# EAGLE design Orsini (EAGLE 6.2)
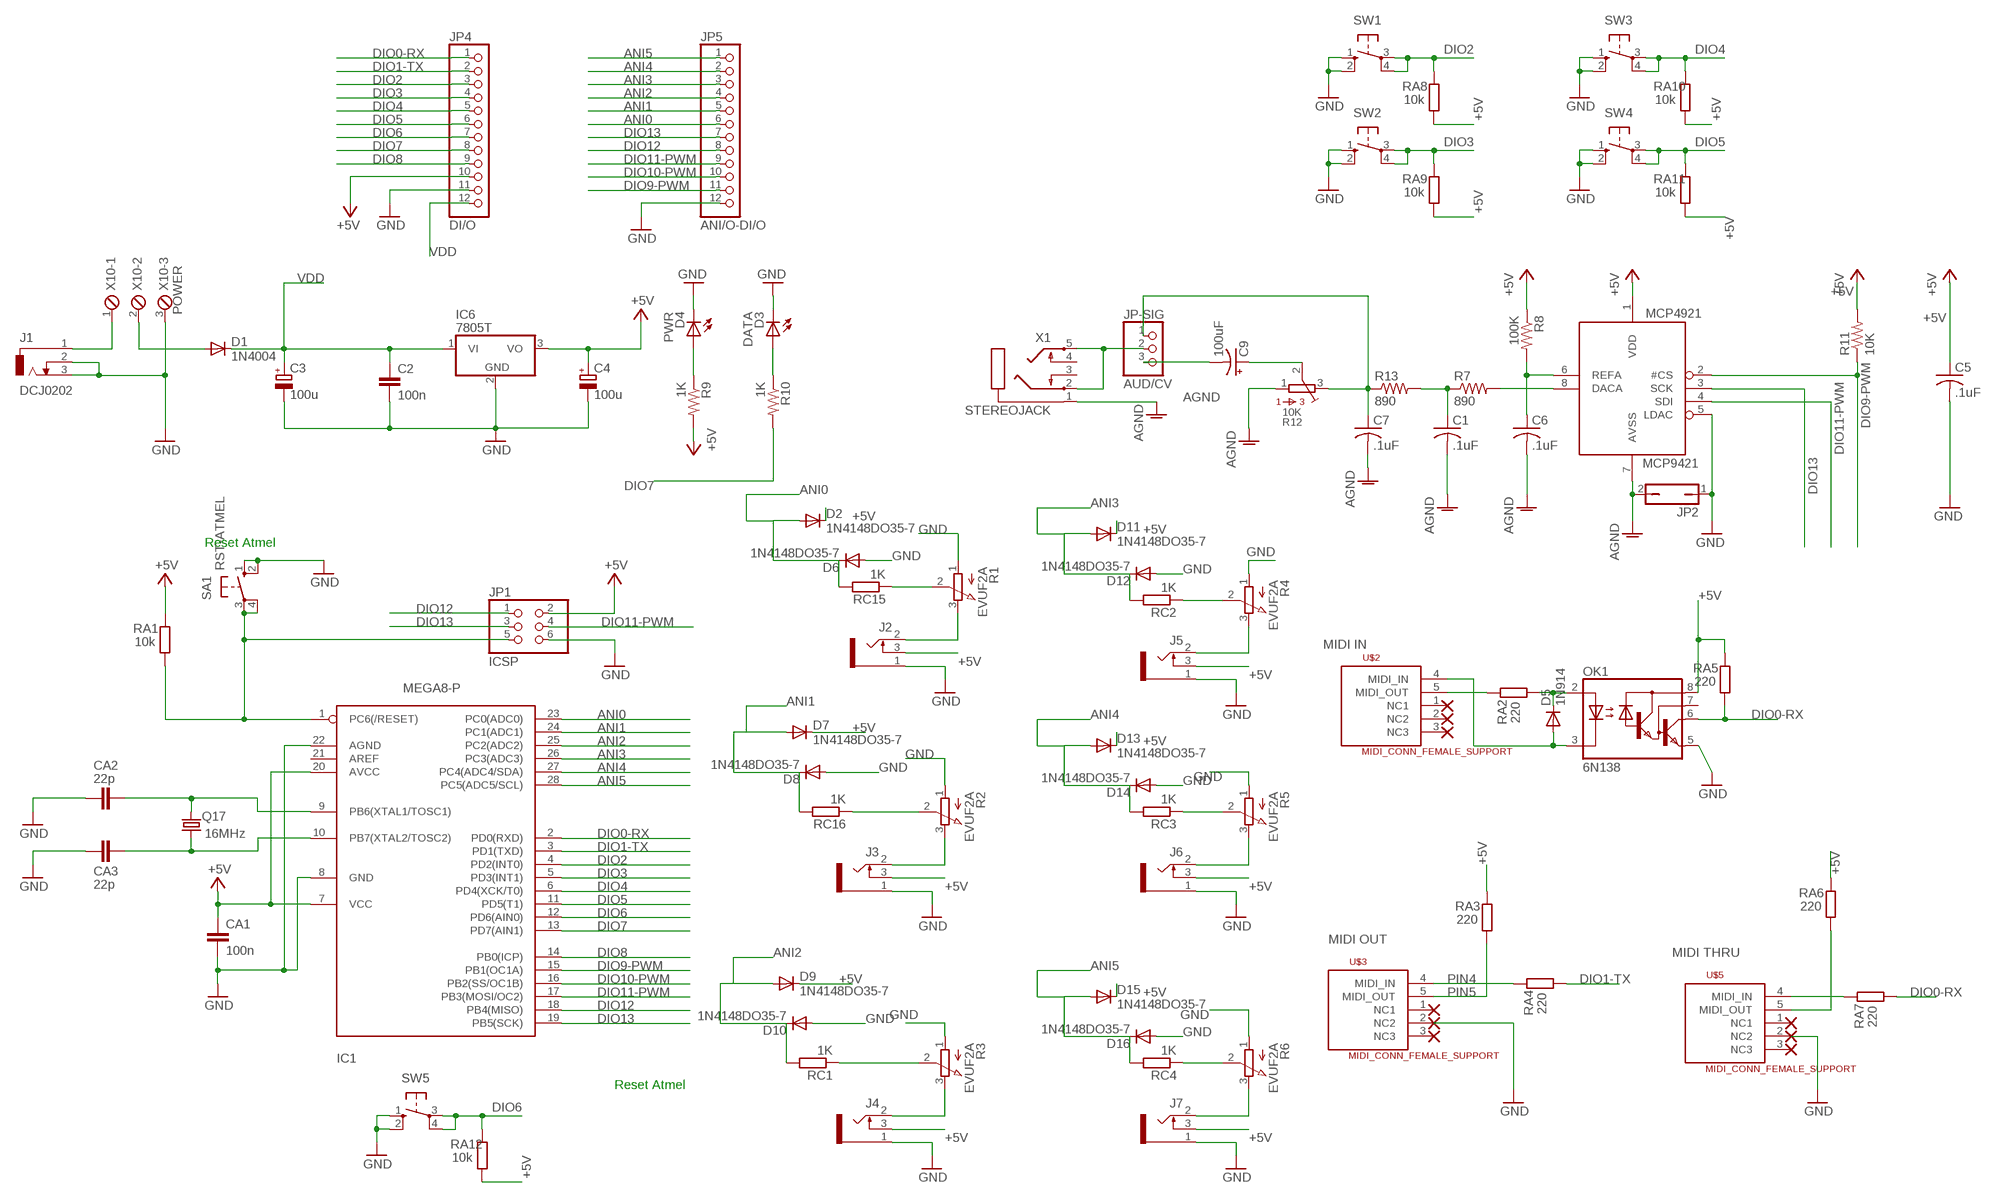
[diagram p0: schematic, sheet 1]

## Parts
C1  .1uF  C-US050-025X075  [C050-025X075]
C2  100n  C-EU050-025X075  [C050-025X075]
C3  100u  CPOL-EUE2.5-7  [E2,5-7]
C4  100u  CPOL-EUE2.5-7  [E2,5-7]
C5  .1uF  C-US025-025X050  [C025-025X050]
C6  .1uF  C-US025-025X050  [C025-025X050]
C7  .1uF  C-US050-025X075  [C050-025X075]
C9  100uF  CPOL-USE2.5-5  [E2,5-5]
CA1  100n  C-EU050-025X075  [C050-025X075]
CA2  22p  C-EU050-025X075  [C050-025X075]
CA3  22p  C-EU050-025X075  [C050-025X075]
D1  1N4004  [DO41-10]
D2  1N4148DO35-7  [DO35-7]
D3  DATA  HLMP-M  [LED4MM]
D4  PWR  HLMP-M  [LED4MM]
D5  1N914  BAS15  [DO34-7]
D6  1N4148DO35-7  [DO35-7]
D7  1N4148DO35-7  [DO35-7]
D8  1N4148DO35-7  [DO35-7]
D9  1N4148DO35-7  [DO35-7]
D10  1N4148DO35-7  [DO35-7]
D11  1N4148DO35-7  [DO35-7]
D12  1N4148DO35-7  [DO35-7]
D13  1N4148DO35-7  [DO35-7]
D14  1N4148DO35-7  [DO35-7]
D15  1N4148DO35-7  [DO35-7]
D16  1N4148DO35-7  [DO35-7]
IC1  MEGA8-P  [DIL28-3]
IC6  7805T  [TO220H]
J1  DCJ0202  [DCJ0202]
J2  1502_03SLOTTED  [1502_03_SLOTTED]
J3  1502_03SLOTTED  [1502_03_SLOTTED]
J4  1502_03SLOTTED  [1502_03_SLOTTED]
J5  1502_03SLOTTED  [1502_03_SLOTTED]
J6  1502_03SLOTTED  [1502_03_SLOTTED]
J7  1502_03SLOTTED  [1502_03_SLOTTED]
JP1  ICSP  PINHD-2X3  [2X03]
JP2  JP1Q  [JP1]
JP4  DI/O  PINHD-1X12  [1X12]
JP5  ANI/O-DI/O  PINHD-1X12  [1X12]
JP-SIG  AUD/CV  PINHD-1X3  [1X03]
MCP4921  MCP9421  [DIL08]
OK1  6N138  [DIL08]
Q17  16MHz  CRYSTALHC49S  [HC49/S]
R1  EVUF2A  [EVUF]
R2  EVUF2A  [EVUF]
R3  EVUF2A  [EVUF]
R4  EVUF2A  [EVUF]
R5  EVUF2A  [EVUF]
R6  EVUF2A  [EVUF]
R7  890  R-US_0207/7  [0207/7]
R8  100K  R-US_0207/7  [0207/7]
R9  1K  R-US_0207/7  [0207/7]
R10  1K  R-US_0207/7  [0207/7]
R11  10K  R-US_0207/10  [0207/10]
R12  10K  3386-F  [3386F]
R13  890  R-US_0207/7  [0207/7]
RA1  10k  R-EU_0207/10  [0207/10]
RA2  220  R-EU_0207/10  [0207/10]
RA3  220  R-EU_0207/10  [0207/10]
RA4  220  R-EU_0207/10  [0207/10]
RA5  220  R-EU_0207/10  [0207/10]
RA6  220  R-EU_0207/10  [0207/10]
RA7  220  R-EU_0207/10  [0207/10]
RA8  10k  R-EU_0207/10  [0207/10]
RA9  10k  R-EU_0207/10  [0207/10]
RA10  10k  R-EU_0207/10  [0207/10]
RA11  10k  R-EU_0207/10  [0207/10]
RA12  10k  R-EU_0207/10  [0207/10]
RC1  1K  R-EU_0207/10  [0207/10]
RC2  1K  R-EU_0207/10  [0207/10]
RC3  1K  R-EU_0207/10  [0207/10]
RC4  1K  R-EU_0207/10  [0207/10]
RC15  1K  R-EU_0207/10  [0207/10]
RC16  1K  R-EU_0207/10  [0207/10]
SA1  RST-ATMEL  10-XX  [B3F-10XX]
SW1  40-XX  [B3F-40XX]
SW2  40-XX  [B3F-40XX]
SW3  40-XX  [B3F-40XX]
SW4  40-XX  [B3F-40XX]
SW5  40-XX  [B3F-40XX]
U$2  MIDI_CONN_FEMALE_SUPPORT  [DIN_5_FEMALE_SUPPORT]
U$3  MIDI_CONN_FEMALE_SUPPORT  [DIN_5_FEMALE_SUPPORT]
U$5  MIDI_CONN_FEMALE_SUPPORT  [DIN_5_FEMALE_SUPPORT]
X1  STEREOJACK  [STX3001]
X10  POWER  MPT3  [3POL254]

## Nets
56: D5.C OK1.2(A) RA2.2
1235: RA3.2 U$3.5(MIDI_OUT)
+5V [Power]: C4.+ C5.1 CA1.1 D2.C D7.C D9.C D11.C D13.C D15.C IC1.7(VCC) IC1.20(AVCC) IC6.3(VO) J2.3 J3.3 J4.3 J5.3 J6.3 J7.3 JP1.2 JP4.10 MCP4921.1(VDD) OK1.8(VCC) R8.1 R9.2 R11.2 RA1.1 RA3.1 RA5.1 RA6.1 RA8.2 RA9.2 RA10.2 RA11.2 RA12.2
AGND [AGND]: C1.2 C6.2 C7.2 JP2.2 MCP4921.7(AVSS) R12.1 X1.1
ANI0: D2.A D6.C IC1.23(PC0(ADC0)) JP5.6 RC15.2
ANI1: D7.A D8.C IC1.24(PC1(ADC1)) JP5.5 RC16.2
ANI2: D9.A D10.C IC1.25(PC2(ADC2)) JP5.4 RC1.2
ANI3: D11.A D12.C IC1.26(PC3(ADC3)) JP5.3 RC2.2
ANI4: D13.A D14.C IC1.27(PC4(ADC4/SDA)) JP5.2 RC3.2
ANI5: D15.A D16.C IC1.28(PC5(ADC5/SCL)) JP5.1 RC4.2
DIO0-RX: IC1.2(PD0(RXD)) JP4.1 OK1.6(VO) RA5.2 RA7.2
DIO1-TX: IC1.3(PD1(TXD)) JP4.2 RA4.2
DIO2: IC1.4(PD2(INT0)) JP4.3 RA8.1 SW1.3(P) SW1.4(P1)
DIO3: IC1.5(PD3(INT1)) JP4.4 RA9.1 SW2.3(P) SW2.4(P1)
DIO4: IC1.6(PD4(XCK/T0)) JP4.5 RA10.1 SW3.3(P) SW3.4(P1)
DIO5: IC1.11(PD5(T1)) JP4.6 RA11.1 SW4.3(P) SW4.4(P1)
DIO6: IC1.12(PD6(AIN0)) JP4.7 RA12.1 SW5.3(P) SW5.4(P1)
DIO7: IC1.13(PD7(AIN1)) JP4.8 R10.2
DIO8: IC1.14(PB0(ICP)) JP4.9
DIO9-PWM: IC1.15(PB1(OC1A)) JP5.11 MCP4921.2(#CS) R11.1
DIO10-PWM: IC1.16(PB2(SS/OC1B)) JP5.10
DIO11-PWM: IC1.17(PB3(MOSI/OC2)) JP1.4 JP5.9 MCP4921.4(SDI)
DIO12: IC1.18(PB4(MISO)) JP1.1 JP5.8
DIO13: IC1.19(PB5(SCK)) JP1.3 JP5.7 MCP4921.3(SCK)
GND [GND]: C2.2 C3.- C4.- C5.2 CA1.2 CA2.2 CA3.2 D3.A(C) D4.A(C) D6.A D8.A D10.A D12.A D14.A D16.A IC1.8(GND) IC1.22(AGND) IC6.2(GND) J1.2 J1.3 J2.1 J3.1 J4.1 J5.1 J6.1 J7.1 JP1.6 JP2.1 JP4.11 JP5.12 MCP4921.5(LDAC) OK1.5(GND) R1.1(A) R2.1(A) R3.1(A) R4.1(A) R5.1(A) R6.1(A) SA1.1(S) SA1.2(S1) SW1.1(S) SW1.2(S1) SW2.1(S) SW2.2(S1) SW3.1(S) SW3.2(S1) SW4.1(S) SW4.2(S1) SW5.1(S) SW5.2(S1) U$3.2(NC2) U$5.2(NC2) X10.3
N$1: J1.1 X10.1
N$2: IC1.1(PC6(/RESET)) JP1.5 RA1.2 SA1.3(P) SA1.4(P1)
N$3: R1.2(S) RC15.1
N$4: D1.A X10.2
N$5: CA2.1 IC1.9(PB6(XTAL1/TOSC1)) Q17.2
N$6: CA3.1 IC1.10(PB7(XTAL2/TOSC2)) Q17.1
N$7: J2.2 R1.3(E)
N$8: RA4.1 U$3.4(MIDI_IN)
N$9: RA6.2 U$5.5(MIDI_OUT)
N$10: R2.2(S) RC16.1
N$11: J3.2 R2.3(E)
N$12: R3.2(S) RC1.1
N$13: RA7.1 U$5.4(MIDI_IN)
N$14: RA2.1 U$2.5(MIDI_OUT)
N$15: MCP4921.8(DACA) R7.2
N$16: JP-SIG.2 X1.2 X1.5
N$17: C7.1 JP-SIG.1 R12.3 R13.1
N$18: C6.1 MCP4921.6(REFA) R8.2
N$19: C1.1 R7.1 R13.2
N$20: C9.- JP-SIG.3
N$21: D3.K(A) R10.1
N$22: J4.2 R3.3(E)
N$23: R4.2(S) RC2.1
N$24: R5.2(S) RC3.1
N$25: D4.K(A) R9.1
N$26: J5.2 R4.3(E)
N$27: J6.2 R5.3(E)
N$28: J7.2 R6.3(E)
N$29: R6.2(S) RC4.1
N$42: C9.+ R12.2
PIN5: D5.A OK1.3(C) U$2.4(MIDI_IN)
VDD [Power]: C2.1 C3.+ D1.C IC6.1(VI) JP4.12
Unconnected: IC1.21(AREF) OK1.7(VB) U$2.1(NC1) U$2.2(NC2) U$2.3(NC3) U$3.1(NC1) U$3.3(NC3) U$5.1(NC1) U$5.3(NC3) X1.3 X1.4

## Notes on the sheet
- Reset Atmel
- MIDI IN
- MIDI OUT
- MIDI THRU
- PIN4
- PIN5
- Reset Atmel

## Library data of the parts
C1 C5-C7 = CMC:C-US: CAPACITOR, American symbol
C2 CA1-CA3 = rcl:C-EU: CAPACITOR, European symbol
C3 C4 = rcl:CPOL-EU: POLARIZED CAPACITOR, European symbol
C9 = rcl-ez:CPOL-US: POLARIZED CAPACITOR, American symbol
D1 = diode:1N4004: DIODE
D2 D6-D16 = diode:1N4148: DIODE
D3 D4 = CMC:HLMP-M: 4mm Flat Top LED
D5 = diode:BAS15: DIODE
IC1 = atmel:MEGA8-P: MICROCONTROLLER 8 Kbytes FLASH, 1 kbytes SRAM, 512 bytes EEPROM, USART, 4-channel 10 bit ADC, 2-channel 8 bit ADC Pin compatible with Atmega48, ATMega88, ATMega168 Source: avr.lbr
IC6 = linear:78*: Positive VOLTAGE REGULATOR Source: http://cache.national.com/ds/LM/LM78L05.pdf http://www.fairchildsemi.com/ds/LM/LM7805.pdf
J1 = con-jack:DCJ0202: DC POWER JACK Source: DCJ0202.pdf
J2-J7 = og-lumberg:1502_03
JP1 = pinhead:PINHD-2X3: PIN HEADER
JP2 = jumper:JP1Q: JUMPER
JP4 JP5 = pinhead:PINHD-1X12: PIN HEADER
JP-SIG = pinhead:PINHD-1X3: PIN HEADER
MCP4921 = ashield:MCP9421
OK1 = optocoupler:6N138: MOTOROLA OPTO COUPLER; MF: VISHAY/TELEFUNKEN; MPN: 6N138; OC_FARNELL: 9860150; OC_NEWARK: 35K5294
Q17 = crystal:CRYSTAL: CRYSTAL
R1-R6 = pot:EVU: 9 mm Square Rotary Potentiometers Source: Panasonic
R7-R11 R13 = rcl-ez:R-US_: RESISTOR, American symbol
R12 = BOURNS:3386-: 3386 Series 3/8" Square Trimmer
RA1-RA12 RC1-RC4 RC15 RC16 = rcl:R-EU_: RESISTOR, European symbol
SA1 = switch-omron:10-XX: OMRON SWITCH
SW1-SW5 = og-switch:40-XX: OMRON SWITCH
U$2 U$3 U$5 = SparkFun:MIDI_CONN_FEMALE_SUPPORT
X1 = ashield:STEREOJACK: MIC/HEADPHONE JACK KS-S stereo microphone/headphone jack PG203JN (Schukat)
X10 = con-phoenix-254:MPT3: PHOENIX CONNECTOR

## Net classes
0 default: width 0.406 mm, drill 0.508 mm, clearance 0.305 mm
1 GND: width 0.61 mm, drill 0.508 mm, clearance 0.305 mm
2 Power: width 0.61 mm, drill 0.508 mm, clearance 0.305 mm
3 AGND: width 0.61 mm, drill 0.508 mm, clearance 0.305 mm

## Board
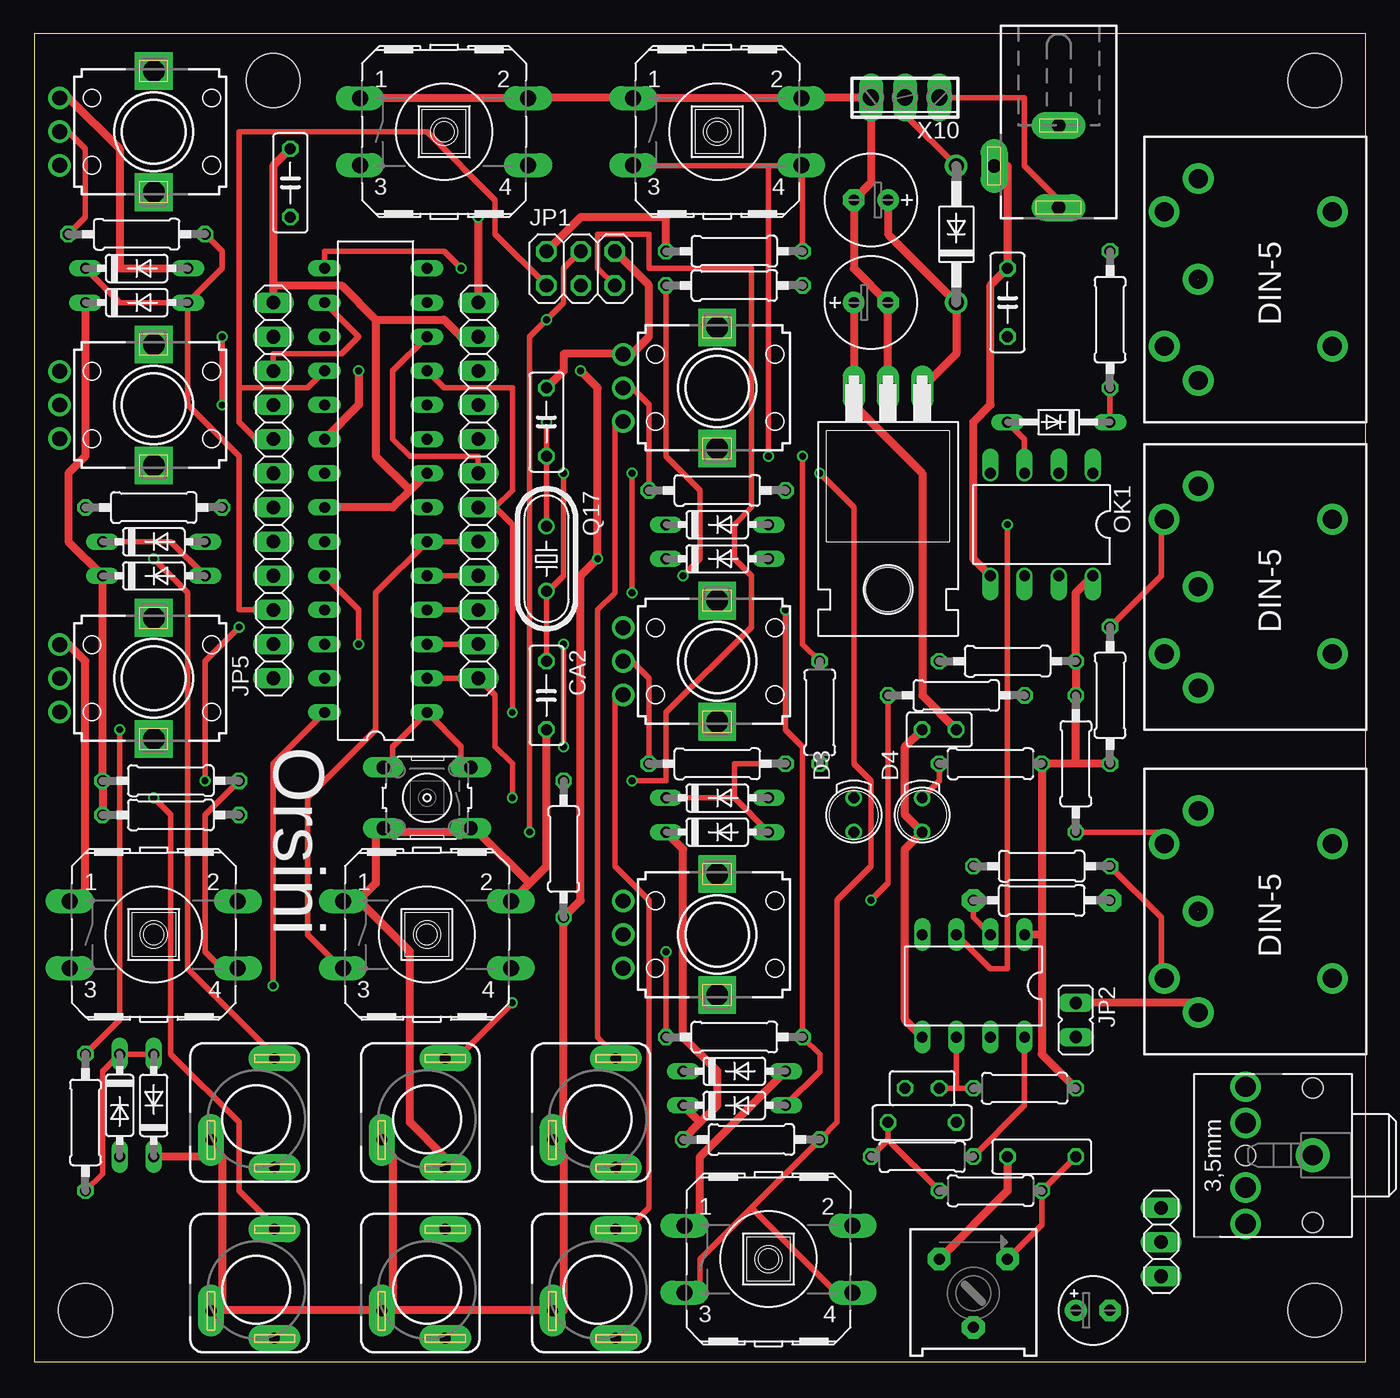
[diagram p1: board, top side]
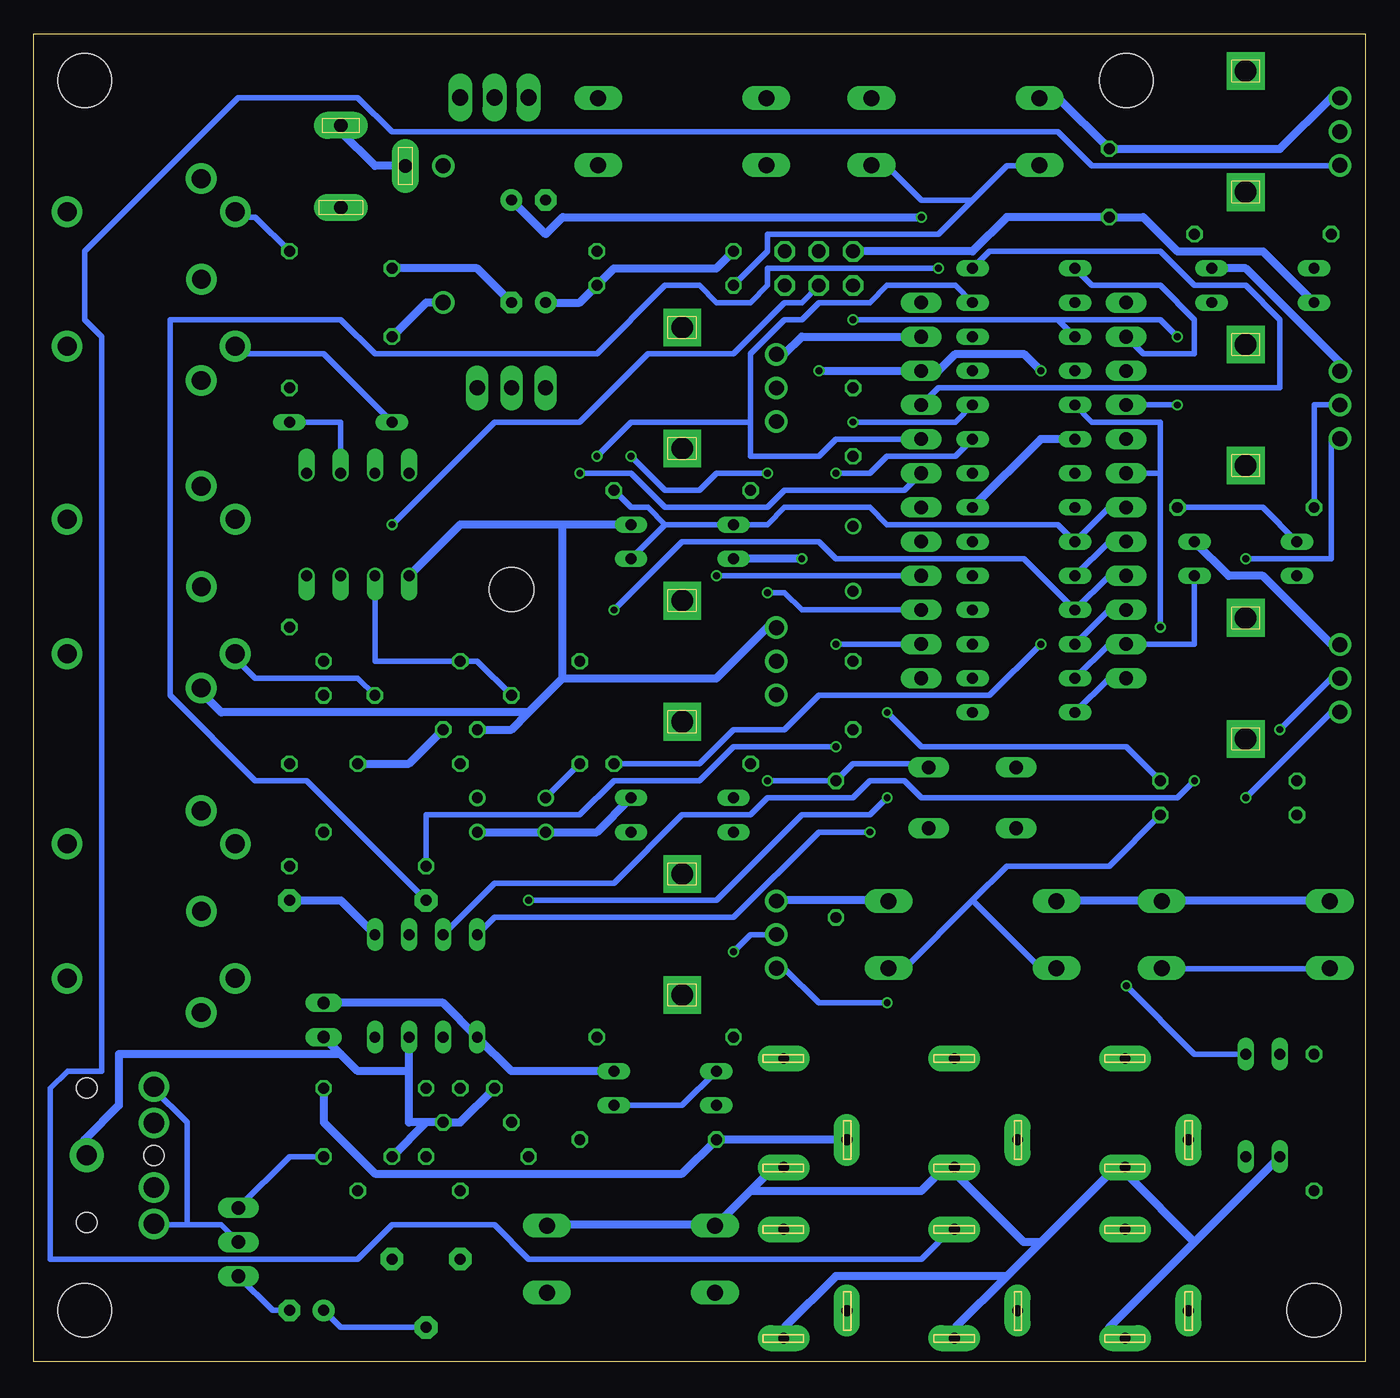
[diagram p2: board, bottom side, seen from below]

Size 99.04 x 98.73 mm. Coordinates in mm from the lower left corner, seen from the top.
Outline: 0,0 99.04,0 99.04,98.73 0,98.73 0,0
Copper layers (1*2*15*16): Top 0.035mm / dielectric 0.2mm / Route2 0.0175mm / dielectric 1.1mm / Route15 0.0175mm / dielectric 0.2mm / Bottom 0.035mm
Design rules: minimum track width 6mil, minimum drill 12mil, track to track 6mil, track to pad 6mil, pad to pad 6mil, via to via 6mil, smd to smd 0mil, copper to edge 10mil, drill to drill 10mil, minimum pad ring 6mil, minimum via ring 6mil, stop-mask expansion 2mil, vias tented up to drill 25mil, thermal gap 10mil
Holes 4 mm at 17.78,95.25 95.25,95.25 95.25,3.81 3.81,3.81

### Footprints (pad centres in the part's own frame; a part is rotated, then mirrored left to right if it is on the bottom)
C050-025X075 = drill 0.813 octagon: 1 -2.54,0; 2 2.54,0
E2,5-7 = drill 0.813 pad 1.6: + -1.27,0 | drill 0.813 pad 1.6 octagon: - 1.27,0
C025-025X050 = drill 0.813 octagon: 1 -1.27,0; 2 1.27,0
E2,5-5 = drill 0.813 pad 1.6: + -1.27,0 | drill 0.813 pad 1.6 octagon: - 1.27,0
DO41-10 = drill 1.118: A 5.08,0; C -5.08,0
DO35-7 = drill 0.813 long: A 3.81,0; C -3.81,0
LED4MM = drill 0.813: A -1.27,0; K 1.27,0
DO34-7 = drill 0.813 long: A 3.81,0; C -3.81,0
DIL28-3 = drill 0.813 long: 1 -16.51,-3.81; 2 -13.97,-3.81; 3 -11.43,-3.81; 4 -8.89,-3.81; 5 -6.35,-3.81; 6 -3.81,-3.81; 7 -1.27,-3.81; 8 1.27,-3.81; 9 3.81,-3.81; 10 6.35,-3.81; 11 8.89,-3.81; 12 11.43,-3.81; 13 13.97,-3.81; 14 16.51,-3.81; 15 16.51,3.81; 16 13.97,3.81; 17 11.43,3.81; 18 8.89,3.81; 19 6.35,3.81; 20 3.81,3.81; 21 1.27,3.81; 22 -1.27,3.81; 23 -3.81,3.81; 24 -6.35,3.81; 25 -8.89,3.81; 26 -11.43,3.81; 27 -13.97,3.81; 28 -16.51,3.81
TO220H = drill 1.118 long: 1 -2.54,-10.16; 2 0,-10.16; 3 2.54,-10.16 | hole 3.302: 0,4.826
DCJ0202 = drill 1 pad 2 long: 1 0,3.1; 2 4.8,0; 3 0,-3
1502_03_SLOTTED = drill 0.8 pad 1.93 long: 1 1.35,-3.34; 2 1.35,4.76; 3 -3.35,-1.29
2X03 = drill 1.016 octagon: 1 -2.54,-1.27; 2 -2.54,1.27; 3 0,-1.27; 4 0,1.27; 5 2.54,-1.27; 6 2.54,1.27
JP1 = drill 0.914 long: 1 0,-1.27; 2 0,1.27
1X12 = drill 1.016 long: 1 -13.97,0; 2 -11.43,0; 3 -8.89,0; 4 -6.35,0; 5 -3.81,0; 6 -1.27,0; 7 1.27,0; 8 3.81,0; 9 6.35,0; 10 8.89,0; 11 11.43,0; 12 13.97,0
1X03 = drill 1.016 long: 1 -2.54,0; 2 0,0; 3 2.54,0
DIL08 = drill 0.813 long: 1 -3.81,-3.81; 2 -1.27,-3.81; 3 1.27,-3.81; 4 3.81,-3.81; 5 3.81,3.81; 6 1.27,3.81; 7 -1.27,3.81; 8 -3.81,3.81
DIL08' = drill 0.813 offset: 1 -3.81,-3.81; 2 -1.27,-3.81; 3 1.27,-3.81; 4 3.81,-3.81; 5 3.81,3.81; 6 1.27,3.81; 7 -1.27,3.81; 8 -3.81,3.81
HC49/S = drill 0.813: 1 -2.413,0; 2 2.413,0
EVUF = drill 1.1 pad 1.676: 1 -2.5,-7; 2 0,-7; 3 2.5,-7 | drill 1.6 pad 2.8 square: M1 4.5,0; M2 -4.5,0
0207/7 = drill 0.813 octagon: 1 -3.81,0; 2 3.81,0
0207/10 = drill 0.813 pad 1.676 octagon: 1 -5.08,0; 2 5.08,0
3386F = drill 0.813 pad 1.676 octagon: 1 -2.54,2.54; 2 0,-2.54; 3 2.54,2.54
0207/10' = drill 0.813 octagon: 1 -5.08,0; 2 5.08,0
B3F-10XX = drill 1.016 long: 1 -3.251,2.261; 2 3.251,2.261; 3 -3.251,-2.261; 4 3.251,-2.261
B3F-40XX = drill 1.194 long: 1 -6.248,2.489; 2 6.248,2.489; 3 -6.248,-2.489; 4 6.248,-2.489
DIN_5_FEMALE_SUPPORT = drill 1.4 pad 2.286: 1 0.46,3.61; 2 -7.07,3.6; 3 7.94,3.6; 4 -4.53,6.12; 5 5.47,6.13; 6 -4.53,-6.382; 7 5.478,-6.382
STX3001 = drill 1.5 pad 2.54: 1 2.7,-0.1 | drill 1.5: 2 7.7,5; 3 7.7,2.3; 4 7.7,-2.5; 5 7.7,-5.2 | hole 1.5: 2.7,4.9; 2.7,-5.1; 7.7,-0.1
3POL254 = drill 1.2 long: 1 -2.54,0; 2 0,0; 3 2.54,0

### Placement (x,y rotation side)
C1  66.04,17.78 0 top
C2  72.39,78.74 90 top
C3  62.23,86.36 180 top
C4  62.23,78.74 0 top
C5  67.31,46.99 180 top
C6  66.04,20.32 180 top
C7  74.93,15.24 180 top
C9  78.74,3.81 0 top
CA1  19.05,87.63 90 top
CA2  38.1,49.53 270 top
CA3  38.1,69.85 90 top
D1  68.58,83.82 90 top
D2  50.8,59.69 0 top
D3  60.96,40.64 90 top
D4  66.04,40.64 90 top
D5  76.2,69.85 180 top
D6  50.8,62.23 0 top
D7  50.8,39.37 0 top
D8  50.8,41.91 0 top
D9  52.07,19.05 0 top
D10  52.07,21.59 0 top
D11  7.62,78.74 0 top
D12  7.62,81.28 0 top
D13  8.89,58.42 0 top
D14  8.89,60.96 0 top
D15  8.89,19.05 90 top
D16  6.35,19.05 270 top
IC1  25.4,64.77 90 top
IC6  63.5,62.23 180 top
J1  76.2,88.9 180 top
J2  41.91,17.78 0 top
J3  41.91,5.08 0 top
J4  29.21,17.78 0 top
J5  29.21,5.08 0 top
J6  16.51,17.78 0 top
J7  16.51,5.08 0 top
JP1  40.64,81.28 0 top
JP2  77.47,25.4 180 top
JP4  33.02,64.77 90 top
JP5  17.78,64.77 90 top
JP-SIG  83.82,8.89 270 top
MCP4921  69.85,27.94 180 top
OK1  6N138  [DIL08']  74.93,62.23 180 top
Q17  38.1,59.69 270 top
R1  50.8,72.39 270 top
R2  50.8,52.07 270 top
R3  50.8,31.75 270 top
R4  8.89,91.44 270 top
R5  8.89,71.12 270 top
R6  8.89,50.8 270 top
R7  66.04,15.24 0 top
R8  73.66,20.32 180 top
R9  71.12,44.45 0 top
R10  58.42,48.26 90 top
R11  74.93,34.29 0 top
R12  69.85,5.08 0 top
R13  71.12,12.7 180 top
RA1  10k  [0207/10']  39.37,38.1 90 top
RA2  220  [0207/10']  80.01,77.47 270 top
RA3  220  [0207/10']  77.47,44.45 270 top
RA4  220  [0207/10']  74.93,36.83 180 top
RA5  220  [0207/10']  72.39,52.07 180 top
RA6  220  [0207/10']  80.01,49.53 90 top
RA7  220  [0207/10']  68.58,49.53 180 top
RA8  10k  [0207/10']  52.07,82.55 180 top
RA9  10k  [0207/10']  52.07,80.01 0 top
RA10  10k  [0207/10']  10.16,40.64 180 top
RA11  10k  [0207/10']  10.16,43.18 180 top
RA12  10k  [0207/10']  53.34,16.51 180 top
RC1  1K  [0207/10']  52.07,24.13 0 top
RC2  1K  [0207/10']  7.62,83.82 0 top
RC3  1K  [0207/10']  8.89,63.5 0 top
RC4  1K  [0207/10']  3.81,17.78 270 top
RC15  1K  [0207/10']  50.8,64.77 0 top
RC16  1K  [0207/10']  50.8,44.45 0 top
SA1  29.21,41.91 180 top
SW1  50.8,91.44 0 top
SW2  30.48,91.44 0 top
SW3  29.21,31.75 0 top
SW4  8.89,31.75 0 top
SW5  54.61,7.62 0 top
U$2  90.17,80.01 90 top
U$3  90.17,33.02 90 top
U$5  90.17,57.15 90 top
X1  97.79,15.24 180 top
X10  64.77,93.98 180 top

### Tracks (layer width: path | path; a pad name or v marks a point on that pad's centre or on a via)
56
  Top 0.406: D5.C RA2.2
  Bottom 0.406: OK1.2 76.2,69.85 D5.C
1235
  Top 0.406: RA3.2 83.82,39.37 U$3.5
+5V  (via drill 0.51)
  Top 0.61: D7.C 48.26,38.1 48.26,24.13 50.8,21.59 50.8,19.05 49.53,17.78 | RA12.2 49.53,17.78 | 49.53,17.78 D9.C | D15.C 12.7,15.24 J6.3 13.97,15.24 13.97,3.81 | 26.67,3.81 26.67,15.24 J4.3 | v40.64,73.66 41.91,72.39 v41.91,59.69 40.64,58.42 40.64,34.29 RA1.1 39.37,16.51 J2.3 39.37,15.24 39.37,3.81 J3.3 38.1,3.81 26.67,3.81 | IC1.20 24.13,71.12 v24.13,73.66 | 26.67,3.81 J5.3 25.4,3.81 13.97,3.81 | 13.97,3.81 J7.3 | OK1.8 77.47,57.15 RA5.1 RA3.1 77.47,44.45 | RA6.1 77.47,44.45 | 77.47,44.45 R9.2 74.93,31.75 | R8.1 74.93,22.86 74.93,31.75 | 74.93,31.75 MCP4921.1 | JP1.2 40.64,85.09 46.99,85.09 RA8.2 | C4.+ IC6.3 60.96,71.12 66.04,66.04 66.04,49.53 C5.1 | RA10.2 RA11.2 D13.C 2.54,60.96 2.54,66.04 3.81,67.31 D11.C
  Bottom 0.61: IC1.7 24.13,68.58 IC1.20 | v41.91,59.69 D2.C | v40.64,73.66 JP4.10 31.75,73.66 30.48,74.93 25.4,74.93 v24.13,73.66 | J2.3 39.37,16.51 RA12.2 50.8,13.97 73.66,13.97 77.47,17.78 R8.1 | MCP4921.1 76.2,34.29 R11.2 | C5.1 71.12,44.45 R9.2 | C4.+ 58.42,78.74 RA9.2 55.88,81.28 48.26,81.28 RA8.2 | D11.C 7.62,82.55 13.97,82.55 16.51,85.09 CA1.1 26.67,85.09 29.21,82.55 JP1.2
AGND
  Top 0.61: R12.1 72.39,12.7 C7.2
  Bottom 0.61: 69.85,17.78 C7.2 | 69.85,17.78 C1.2 67.31,17.78 C6.2 | 71.12,21.59 71.12,17.78 69.85,17.78 | 71.12,21.59 MCP4921.7 | 76.2,22.86 74.93,21.59 71.12,21.59 | 76.2,22.86 JP2.2 | 76.2,22.86 92.71,22.86 92.71,19.05 95.25,16.51 X1.1
ANI0
  Bottom 0.406: JP5.6 19.05,63.5 IC1.23 22.86,62.23 35.56,62.23 36.83,63.5 43.18,63.5 44.45,62.23 D6.C 52.07,62.23 | 52.07,62.23 D2.A | RC15.2 54.61,63.5 53.34,63.5 52.07,62.23
ANI1  (via drill 0.51)
  Top 0.406: 52.07,41.91 D8.C | D7.A 52.07,41.91 | RC16.2 52.07,44.45 52.07,41.91 | IC1.24 24.13,55.88 v24.13,53.34
  Bottom 0.406: IC1.24 19.05,60.96 JP5.5 | v24.13,53.34 27.94,49.53 40.64,49.53 43.18,46.99 46.99,46.99 49.53,44.45 RC16.2
ANI2  (via drill 0.51)
  Top 0.406: D9.A 58.42,21.59 58.42,22.86 RC1.2 57.15,45.72 55.88,46.99 v55.88,55.88
  Bottom 0.406: JP5.4 19.05,58.42 IC1.25 25.4,59.69 39.37,59.69 40.64,60.96 50.8,60.96 v55.88,55.88 | D10.C 50.8,19.05 D9.A
ANI3
  Top 0.406: D11.A 13.97,81.28 13.97,82.55 RC2.2 | D12.C 6.35,78.74 D11.A | JP5.3 15.24,55.88 15.24,67.31 11.43,71.12 D11.A
  Bottom 0.406: IC1.26 19.05,55.88 JP5.3
ANI4
  Top 0.406: D14.C 10.16,60.96 D13.A
  Bottom 0.406: D14.C 7.62,63.5 RC3.2 | D13.A 12.7,53.34 JP5.2 19.05,53.34 IC1.27
ANI5  (via drill 0.51)
  Top 0.406: RC4.2 5.08,13.97 5.08,21.59 D16.C D15.A | IC1.28 17.78,44.45 v17.78,27.94
  Bottom 0.406: IC1.28 19.05,50.8 JP5.1 | v17.78,27.94 12.7,22.86 D15.A
DIO0-RX  (via drill 0.51)
  Top 0.406: IC1.2 JP4.1 34.29,49.53 34.29,45.72 35.56,44.45 v35.56,41.91 | v62.23,34.29 63.5,35.56 RA7.2
  Bottom 0.406: RA7.2 66.04,52.07 RA5.2 73.66,52.07 OK1.6 | v35.56,41.91 36.83,40.64 41.91,40.64 48.26,34.29 v62.23,34.29
DIO1-TX  (via drill 0.51)
  Top 0.406: v39.37,53.34 v39.37,45.72 | JP4.2 IC1.3
  Bottom 0.406: RA4.2 69.85,40.64 58.42,40.64 55.88,43.18 49.53,43.18 46.99,45.72 v39.37,45.72 | JP4.2 v39.37,53.34
DIO2  (via drill 0.51)
  Top 0.406: JP4.3 IC1.4 | RA8.1 57.15,88.9 SW1.4 55.88,88.9 54.61,88.9 | 54.61,88.9 45.72,88.9 SW1.3 | v44.45,66.04 v44.45,57.15 | 54.61,88.9 v54.61,67.31
  Bottom 0.406: JP4.3 41.91,55.88 43.18,57.15 v44.45,57.15 | v44.45,66.04 48.26,66.04 49.53,64.77 52.07,64.77 v54.61,67.31
DIO3  (via drill 0.51)
  Top 0.406: JP4.4 IC1.5 | v48.26,58.42 49.53,59.69 49.53,64.77 46.99,67.31 RA9.1
  Bottom 0.406: RA9.1 44.45,82.55 44.45,83.82 31.75,83.82 29.21,86.36 | 29.21,86.36 26.67,88.9 25.4,88.9 SW2.3 | 29.21,86.36 33.02,86.36 35.56,88.9 SW2.4 | v48.26,58.42 JP4.4
DIO4
  Top 0.406: JP4.5 IC1.6 25.4,57.15 25.4,46.99 20.32,41.91 20.32,31.75 22.86,29.21 SW3.3
  Bottom 0.406: RA10.1 19.05,36.83 26.67,36.83 29.21,34.29 | 29.21,34.29 34.29,29.21 SW3.4 | 29.21,34.29 24.13,29.21 SW3.3
DIO5  (via drill 0.51)
  Top 0.406: IC1.11 30.48,72.39 35.56,72.39 35.56,64.77 34.29,63.5 | RA11.1 12.7,40.64 12.7,30.48 13.97,29.21 SW4.4 | 34.29,63.5 35.56,62.23 v35.56,48.26 | 34.29,63.5 JP4.6
  Bottom 0.406: SW4.3 3.81,29.21 13.97,29.21 SW4.4 | v35.56,48.26 33.02,45.72 17.78,45.72 RA11.1
DIO6  (via drill 0.51)
  Top 0.406: IC1.12 26.67,73.66 26.67,68.58 27.94,67.31 33.02,67.31 JP4.7 | 53.34,11.43 49.53,7.62 49.53,5.08 SW5.3 | 53.34,11.43 RA12.1 59.69,17.78 59.69,34.29 62.23,36.83 62.23,43.18 60.96,44.45 60.96,63.5 v58.42,66.04 | 53.34,11.43 59.69,5.08 SW5.4
  Bottom 0.406: JP4.7 34.29,64.77 43.18,64.77 44.45,63.5 52.07,63.5 54.61,66.04 v58.42,66.04
DIO7  (via drill 0.51)
  Top 0.406: R10.2 57.15,53.34 v57.15,67.31
  Bottom 0.406: IC1.13 30.48,80.01 35.56,80.01 36.83,78.74 40.64,78.74 41.91,77.47 43.18,77.47 45.72,74.93 45.72,69.85 | 45.72,69.85 45.72,67.31 40.64,67.31 39.37,68.58 JP4.8 | v57.15,67.31 54.61,69.85 45.72,69.85
DIO8
  Bottom 0.406: IC1.14 27.94,82.55 15.24,82.55 12.7,80.01 8.89,80.01 6.35,77.47 6.35,72.39 31.75,72.39 JP4.9
DIO9-PWM  (via drill 0.51)
  Top 0.406: MCP4921.2 69.85,33.02 R11.1 | v31.75,81.28 30.48,82.55 21.59,82.55 IC1.15
  Bottom 0.406: IC1.15 20.32,80.01 15.24,80.01 12.7,77.47 12.7,74.93 16.51,74.93 JP5.11 | R11.1 78.74,43.18 82.55,43.18 88.9,49.53 88.9,77.47 76.2,77.47 73.66,74.93 57.15,74.93 52.07,80.01 49.53,80.01 48.26,78.74 45.72,78.74 44.45,80.01 44.45,81.28 v31.75,81.28
DIO10-PWM
  Top 0.406: IC1.16 24.13,76.2 22.86,74.93 17.78,74.93 JP5.10
DIO11-PWM  (via drill 0.51)
  Top 0.406: JP1.4 39.37,81.28 39.37,78.74 v38.1,77.47 36.83,76.2 v36.83,39.37 | v13.97,76.2 v13.97,71.12
  Bottom 0.406: 22.86,77.47 IC1.17 | v38.1,77.47 22.86,77.47 | MCP4921.4 64.77,33.02 46.99,33.02 40.64,39.37 v36.83,39.37 | v13.97,71.12 JP5.9 | v13.97,76.2 15.24,77.47 22.86,77.47
DIO12
  Top 0.406: IC1.18 20.32,72.39 15.24,72.39 | 15.24,72.39 15.24,69.85 16.51,68.58 JP5.8 | JP1.1 34.29,83.82 34.29,86.36 29.21,91.44 15.24,91.44 15.24,72.39
DIO13  (via drill 0.51)
  Top 0.406: MCP4921.3 71.12,29.21 72.39,29.21 v72.39,62.23 | v15.24,54.61 12.7,52.07 v12.7,43.18
  Bottom 0.406: IC1.19 20.32,69.85 15.24,69.85 15.24,66.04 | JP5.7 15.24,66.04 | v72.39,62.23 64.77,69.85 58.42,69.85 53.34,74.93 46.99,74.93 43.18,78.74 41.91,78.74 JP1.3 | v15.24,54.61 15.24,66.04 | v12.7,43.18 13.97,41.91 33.02,41.91 34.29,43.18 36.83,43.18 38.1,41.91 44.45,41.91 45.72,40.64 50.8,40.64 55.88,35.56 64.77,35.56 MCP4921.3
GND
  Top 0.61: J1.2 72.39,88.9 C2.2 71.12,80.01 71.12,71.12 69.85,69.85 69.85,59.69 OK1.5 | IC6.2 C4.- 60.96,81.28 C3.- 62.23,87.63 X10.3 57.15,93.98 SW1.2 55.88,93.98 45.72,93.98 SW1.1 44.45,93.98 36.83,93.98 SW2.2 35.56,93.98 25.4,93.98 SW2.1 | CA3.2 39.37,73.66 39.37,74.93 43.18,74.93 R1.1 44.45,74.93 45.72,76.2 45.72,80.01 JP1.6 | IC1.22 26.67,63.5 27.94,64.77 | IC1.8 27.94,64.77 | 17.78,80.01 17.78,88.9 CA1.2 | 17.78,80.01 JP5.12 | 27.94,64.77 25.4,67.31 25.4,77.47 | 25.4,77.47 22.86,80.01 17.78,80.01 | D12.A 6.35,81.28 6.35,90.17 2.54,93.98 R4.1 | JP4.11 31.75,76.2 30.48,77.47 25.4,77.47 | CA2.2 38.1,36.83 36.83,35.56 | 36.83,35.56 35.56,34.29 SW3.2 | 24.13,34.29 25.4,35.56 25.4,39.37 SA1.2 26.67,39.37 31.75,39.37 SA1.1 33.02,39.37 36.83,35.56 | R6.1 2.54,53.34 3.81,52.07 3.81,34.29 SW4.1 | C5.2 64.77,45.72 64.77,40.64 D4.A 64.77,38.1 64.77,25.4 MCP4921.5 | JP2.1 86.36,26.67 U$3.2 | D10.A 49.53,15.24 49.53,10.16 SW5.1 | 24.13,34.29 27.94,30.48 27.94,17.78 30.48,15.24 J4.1 | 24.13,34.29 SW3.1
  Bottom 0.61: J1.2 73.66,88.9 76.2,91.44 J1.3 | C2.2 66.04,81.28 C4.- | JP4.11 41.91,76.2 43.18,74.93 R1.1 | D12.A 8.89,81.28 1.27,73.66 R5.1 | SW2.1 24.13,93.98 22.86,93.98 CA1.2 6.35,90.17 2.54,93.98 R4.1 | R3.1 43.18,34.29 35.56,34.29 SW3.2 | D14.A 10.16,58.42 7.62,58.42 2.54,53.34 R6.1 | SW4.1 3.81,34.29 13.97,34.29 SW4.2 15.24,34.29 22.86,34.29 SW3.1 | OK1.5 67.31,62.23 59.69,62.23 | D6.A 59.69,62.23 | D4.A D3.A 57.15,39.37 D8.A | 59.69,50.8 48.26,50.8 44.45,54.61 R2.1 | 62.23,48.26 63.5,46.99 C5.2 | 62.23,48.26 59.69,50.8 | 62.23,48.26 85.09,48.26 86.36,49.53 U$5.2 | 59.69,50.8 59.69,62.23 | 12.7,8.89 19.05,2.54 J7.1 | 12.7,8.89 D16.A | 24.13,8.89 19.05,13.97 J6.1 17.78,13.97 12.7,8.89 | 24.13,8.89 26.67,6.35 | 26.67,6.35 30.48,2.54 J5.1 | 26.67,6.35 39.37,6.35 43.18,2.54 J3.1 | 24.13,8.89 25.4,8.89 30.48,13.97 J4.1 31.75,13.97 33.02,12.7 45.72,12.7 | D10.A 63.5,21.59 MCP4921.5 68.58,26.67 JP2.1 | SW5.2 59.69,10.16 49.53,10.16 SW5.1 48.26,10.16 45.72,12.7 | 45.72,12.7 44.45,13.97 J2.1
N$1
  Top 0.406: X10.1 73.66,93.98 73.66,88.9 76.2,86.36 J1.1
N$2  (via drill 0.51)
  Top 0.406: SA1.4 26.67,44.45 26.67,45.72 IC1.1 31.75,45.72 31.75,44.45 SA1.3 | JP1.5 41.91,81.28 41.91,83.82 45.72,83.82 45.72,81.28 53.34,81.28 53.34,63.5 52.07,62.23 52.07,59.69 53.34,58.42 53.34,54.61 46.99,48.26 46.99,43.18 v44.45,43.18
  Bottom 0.406: SA1.3 33.02,44.45 38.1,44.45 RA1.2 v44.45,43.18
N$3
  Top 0.406: RC15.1 45.72,71.12 44.45,72.39 R1.2
N$4
  Top 0.406: D1.A 64.77,92.71 X10.2
N$5  (via drill 0.51)
  Top 0.406: 38.1,57.15 CA2.1 | v39.37,66.04 39.37,58.42 38.1,57.15 | 38.1,57.15 Q17.2
  Bottom 0.406: IC1.9 30.48,67.31 35.56,67.31 36.83,66.04 v39.37,66.04
N$6  (via drill 0.51)
  Top 0.406: Q17.1 CA3.1 v38.1,69.85
  Bottom 0.406: IC1.10 30.48,69.85 v38.1,69.85
N$7
  Top 0.406: R1.3 43.18,69.85 43.18,57.15 41.91,55.88 41.91,24.13 43.18,22.86 J2.2
N$8
  Top 0.406: RA4.1 83.82,33.02 83.82,29.21 U$3.4
N$9
  Top 0.406: RA6.2 83.82,58.42 83.82,62.23 U$5.5
N$10
  Top 0.406: RC16.1 45.72,50.8 44.45,52.07 R2.2
N$11
  Top 0.406: R2.3 43.18,49.53 43.18,36.83 45.72,34.29 45.72,11.43 44.45,10.16 J3.2
N$12  (via drill 0.51)
  Top 0.406: v46.99,30.48 RC1.1
  Bottom 0.406: v46.99,30.48 45.72,31.75 R3.2
N$13
  Bottom 0.406: RA7.1 74.93,50.8 82.55,50.8 83.82,52.07 U$5.4
N$14
  Bottom 0.406: RA2.1 82.55,85.09 83.82,85.09 U$2.5
N$15
  Top 0.406: R7.2 73.66,19.05 MCP4921.8
N$16
  Bottom 0.406: JP-SIG.2 85.09,10.16 87.63,10.16 | 87.63,10.16 90.17,10.16 X1.2 | 87.63,10.16 87.63,17.78 90.17,20.32 X1.5
N$17
  Top 0.406: C7.1 R13.1 74.93,10.16 R12.3
  Bottom 0.406: JP-SIG.1 80.01,15.24 C7.1
N$18
  Top 0.406: R8.2 68.58,20.32 | 68.58,20.32 C6.1 | 68.58,20.32 MCP4921.6
N$19
  Top 0.406: 63.5,16.51 R7.1 | C1.1 63.5,16.51 | 63.5,16.51 R13.2
N$20
  Bottom 0.406: JP-SIG.3 81.28,3.81 C9.-
N$21
  Bottom 0.406: R10.1 D3.K
N$22  (via drill 0.51)
  Top 0.406: v35.56,26.67 31.75,22.86 J4.2
  Bottom 0.406: v35.56,26.67 40.64,26.67 43.18,29.21 R3.3
N$23
  Top 0.406: RC2.1 3.81,85.09 3.81,90.17 2.54,91.44 R4.2
N$24
  Bottom 0.406: RC3.1 3.81,71.12 R5.2
N$25
  Top 0.406: D4.K 67.31,43.18 R9.1
N$26
  Bottom 0.406: R4.3 2.54,88.9 20.32,88.9 22.86,91.44 72.39,91.44 74.93,93.98 83.82,93.98 95.25,82.55 95.25,77.47 93.98,76.2 93.98,21.59 96.52,21.59 97.79,20.32 97.79,7.62 74.93,7.62 72.39,10.16 64.77,10.16 62.23,7.62 33.02,7.62 31.75,8.89 J5.2
N$27  (via drill 0.51)
  Top 0.406: v8.89,59.69 11.43,57.15 11.43,29.21 17.78,22.86 J6.2
  Bottom 0.406: v8.89,59.69 2.54,59.69 2.54,68.58 R5.3
N$28  (via drill 0.51)
  Top 0.406: v8.89,41.91 10.16,40.64 10.16,22.86 15.24,17.78 15.24,12.7 17.78,10.16 J7.2
  Bottom 0.406: v8.89,41.91 2.54,48.26 R6.3
N$29  (via drill 0.51)
  Top 0.406: RC4.1 6.35,25.4 v6.35,46.99
  Bottom 0.406: v6.35,46.99 2.54,50.8 R6.2
N$42
  Bottom 0.406: C9.+ 76.2,2.54 R12.2
PIN5
  Top 0.406: D5.A 73.66,68.58 OK1.3
  Bottom 0.406: D5.A 77.47,74.93 83.82,74.93 U$2.4
VDD  (via drill 0.51)
  Top 0.61: IC6.1 68.58,74.93 D1.C 63.5,83.82 C3.+ | v33.02,85.09 JP4.12
  Bottom 0.61: C2.1 69.85,78.74 D1.C | v33.02,85.09 59.69,85.09 60.96,83.82 C3.+

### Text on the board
tNames: Orsini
